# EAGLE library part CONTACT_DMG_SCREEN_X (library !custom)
The lateral input for the DMG screen.
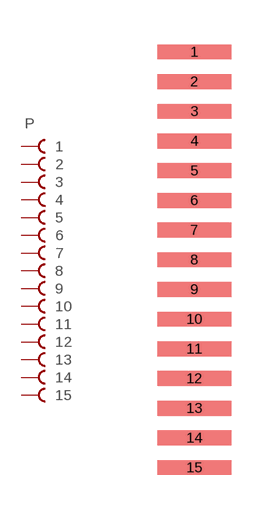
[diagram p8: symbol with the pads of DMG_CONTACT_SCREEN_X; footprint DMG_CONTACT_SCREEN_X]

Designator prefix P

## CONTACT_DMG_SCREEN_X  [DMG_CONTACT_SCREEN_X]
1  1  pas
2  2  pas
3  3  pas
4  4  pas
5  5  pas
6  6  pas
7  7  pas
8  8  pas
9  9  pas
10  10  pas
11  11  pas
12  12  pas
13  13  pas
14  14  pas
15  15  pas

## Footprint DMG_CONTACT_SCREEN_X (pad centres in mm)
smd 2.5 x 0.5: 1 0,7; 2 0,6; 3 0,5; 4 0,4; 5 0,3; 6 0,2; 7 0,1; 8 0,0; 9 0,-1; 10 0,-2; 11 0,-3; 12 0,-4; 13 0,-5; 14 0,-6; 15 0,-7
